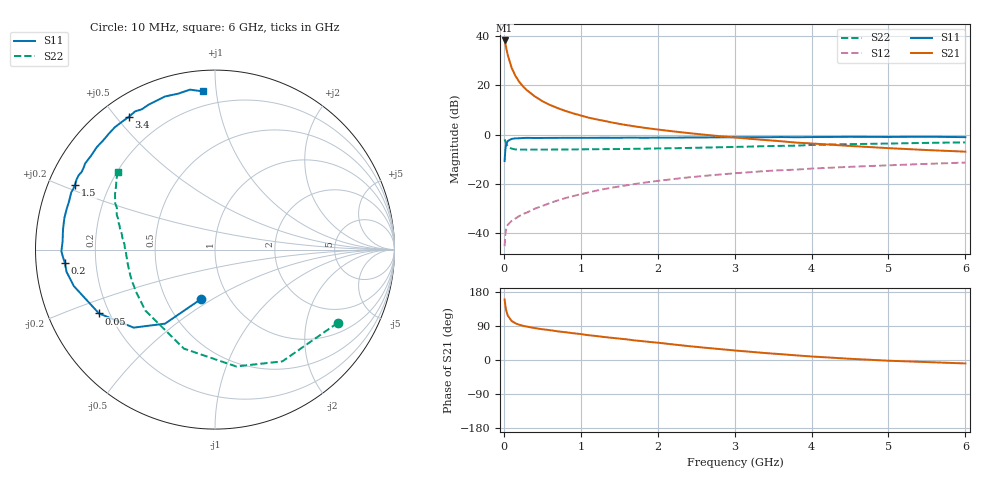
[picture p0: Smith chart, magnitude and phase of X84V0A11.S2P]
! SIEMENS Small Signal Semiconductors
! BFP136W
! Si NPN RF Bipolar Junction Transistor in SOT343
! VCE = 4 V  IC = 110 mA
! Common Emitter S-Parameters:  September  1994
# GHz  S  MA  R  50
!  f  S11  S21  S12  S22
! GHz  MAG  ANG  MAG  ANG  MAG  ANG  MAG  ANG
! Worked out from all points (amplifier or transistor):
!   40 points, 10 MHz to 6 GHz, reference 50 ohm
!   highest |S21| = 38.4 dB at 10 MHz (marker M1)
!   |S21| within 3 dB of that: start of sweep to 30.73 MHz
!   unconditionally stable (mu >= 1): 503.1 MHz to 2.917 GHz
!   at 200 MHz: K = 0.69, MSG = 27.4 dB, |S12| = -33.2 dB
!   at 1.5 GHz: K = 1.10, MAG = 10.8 dB, |S12| = -21.2 dB
!   at 6 GHz: K = 0.98, MSG = 2.2 dB, |S12| = -11.4 dB
!   S11 on the Smith chart (normalised r, x): 10 MHz: 0.74, -0.45; 50 MHz: 0.16, -0.25; 200 MHz: 0.09, -0.04; 1.5 GHz: 0.08, +0.22; 3.4 GHz: 0.08, +0.54; 6 GHz: 0.11, +0.92
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0.01  0.2883 -106.1  82.81 159.9  0.0053 69.3  0.7963 -30.8
0.02  0.4976 -124.0  70.77 143.2  0.0092 56.4  0.7271 -58.9
0.03  0.6282 -136.2  59.37 131.5  0.0116 48.7  0.6618 -79.7
0.05  0.7379 -151.2  42.19 117.5  0.0144 39.0  0.5784 -107.4
0.1  0.8123 -165.5  23.23 103.2  0.0173 37.0  0.5157 -138.9
0.15  0.8365 -171.5  15.8 96.9  0.0194 40.4  0.4987 -151.8
0.2  0.8395 -174.9  11.88 93.1  0.0218 42.0  0.4944 -158.8
0.25  0.8497 -177.6  9.571 90.2  0.024 45.7  0.4933 -163.3
0.3  0.8559 -179.4  8.009 88.1  0.0257 47.7  0.4916 -166.3
0.4  0.8503 176.9  6.029 84.3  0.0307 52.1  0.4926 -170.4
0.5  0.8521 174.3  4.807 81.2  0.035 55.3  0.4932 -173.1
0.6  0.8542 172.3  4.011 78.7  0.0401 57.4  0.4938 -174.9
0.7  0.8556 169.9  3.458 75.6  0.0454 59.3  0.4952 -176.2
0.9  0.8568 166.3  2.706 70.7  0.0556 60.6  0.4971 -178.8
1.1  0.8564 161.7  2.212 65.4  0.0661 61.1  0.5005 179.5
1.5  0.8591 155.3  1.651 56.5  0.0874 60.3  0.5065 176.4
2.2  0.8661 143.1  1.161 41.1  0.1236 55.2  0.525 170.9
3.2  0.8808 126.2  0.818 21.8  0.1707 45.8  0.5676 162.2
3.4  0.8817 123.1  0.773 18.3  0.1802 43.7  0.5806 160.5
4.5  0.8975 108.1  0.586 3.2  0.2197 33.5  0.6375 150.9
5.5  0.9021 98.9  0.483 -5.5  0.2524 25.6  0.6762 144.3
6  0.8843 94.5  0.448 -9.1  0.2684 21.3  0.6916 141.4
